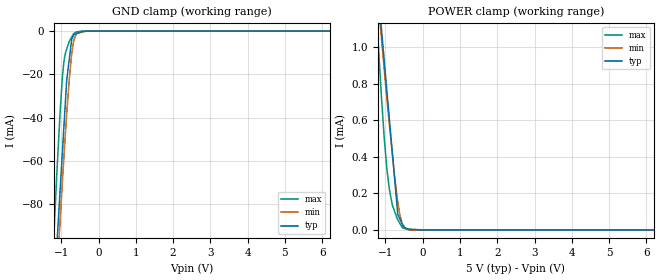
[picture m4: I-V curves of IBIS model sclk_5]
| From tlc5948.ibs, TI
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|   sclk_5 Model
[Model]   sclk_5
Model_type   Input
Vinl = 1.5
Vinh = 3.5
|   typ   min   max
|   (nom PVT)   (fast PVT)   (slow PVT)
|C_comp from frequency sweep method (F=33MHz)
|Average
|C_comp   7.620e-13   7.434e-13   7.862e-13
|C_comp from LC tank measurement(L=1nH)
|Average
|Resonant Frequency(Hz)   6.940e+09   7.080e+09   6.760e+09
C_comp   5.264e-13   5.058e-13   5.549e-13
| Where nom  PVT is Nominal Process, 5V, 90C
|   Fast PVT is Strong Process,  5.5V, -40C
|   Slow PVT is Weak Process,   4.5V, 150C
[Model Spec]
|Subparameter   typ   min   max
Vinl   1.5   1.35   1.65
Vinh   3.5   3.15   3.85
[Voltage Range]   5   4.5   5.5
|Ambient Temperature   25   85   -40
|Junction Temperature
[Temperature Range]   90   150   -40
[Power Clamp Reference]   5   4.5   5.5
[GND Clamp Reference]   0   0   0
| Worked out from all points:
|   GND clamp passes 1 mA (typ) near -0.57 V on its own axis
|   POWER clamp passes 1 mA (typ) near -1.06 V on its own axis
[GND Clamp]
|   Voltage   I(typ)   I(min)   I(max)
-5V       -1.572A    -1.517A    -1.69A
-1.238V   -137.3mA   -151.3mA   -107.9mA
-1.14V    -104.7mA   -120.9mA   -73.16mA
-1.117V   -97.98mA   -113.5mA   -64.88mA
-1.062V   -82.29mA   -96.54mA   -47.32mA
-1.034V   -74.23mA   -88.33mA   -38.29mA
-962.5mV  -53.66mA   -67.39mA   -19.81mA
-907.5mV  -37.83mA   -52.34mA   -11.77mA
-855mV    -22.72mA   -38.3mA    -8.375mA
-720mV    -3.797mA   -10.57mA   -2.748mA
-594mV    -1.187mA   -1.201mA   -371.3uA
10V       0A         0A         0A
[POWER Clamp]
|   Voltage   I(typ)   I(min)   I(max)
-5V       12.85mA    11.04mA    15.23mA
-1.221V   1.415mA    1.312mA    1.114mA
-1.14V    1.176mA    1.126mA    838.7uA
-1.105V   1.096mA    1.047mA    722.3uA
-1.034V   929.8uA    882.4uA    506uA
-968mV    776.6uA    734.1uA    347.5uA
-891mV    598uA      567.1uA    218.4uA
-814mV    419.4uA    413uA      136.3uA
-670mV    85.3uA     153.6uA    55.91uA
-539mV    26.81uA    30.67uA    10.8uA
-229.5mV  3.135uA    95.48nA    29.91nA
10V       0A         0A         0A
